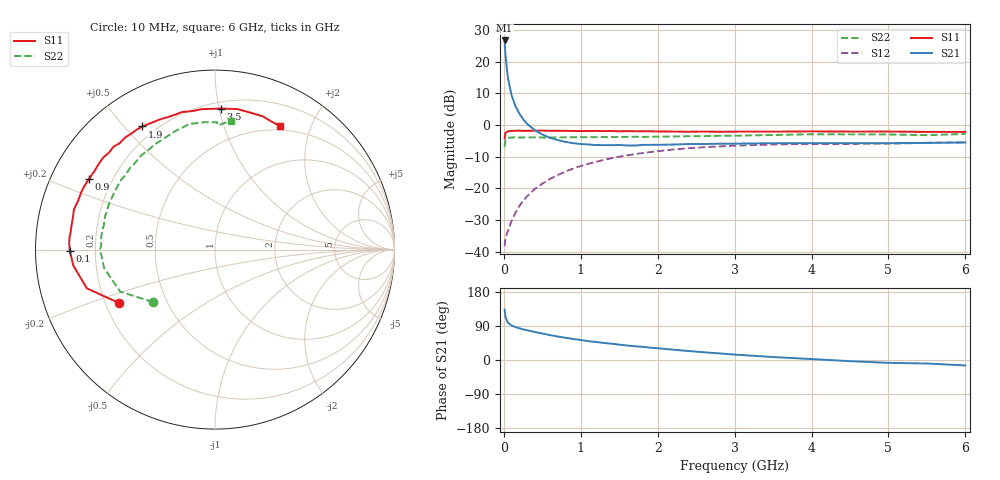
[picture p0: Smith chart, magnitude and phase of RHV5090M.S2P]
! SIEMENS Small Signal Semiconductors
! BFR106
! Si NPN RF Bipolar Junction Transistor in SOT23
! VCE = 0.5 V  IC = 90 mA
! Common Emitter S-Parameters:  August  1996
# GHz  S  MA  R  50
!  f  S11  S21  S12  S22
! GHz  MAG  ANG  MAG  ANG  MAG  ANG  MAG  ANG
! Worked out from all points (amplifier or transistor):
!   36 points, 10 MHz to 6 GHz, reference 50 ohm
!   highest |S21| = 26.7 dB at 10 MHz (marker M1)
!   |S21| within 3 dB of that: start of sweep to 17.19 MHz
!   unconditionally stable (mu >= 1): start of sweep to 17.92 MHz; 25.4 MHz to end of sweep
!   at 250 MHz: K = 1.83, MAG = 7.6 dB, |S12| = -24.0 dB
!   at 1.4 GHz: K = 1.30, MAG = -1.2 dB, |S12| = -10.5 dB
!   at 6 GHz: K = 1.03, MAG = -1.2 dB, |S12| = -5.5 dB
!   S11 on the Smith chart (normalised r, x): 10 MHz: 0.26, -0.24; 100 MHz: 0.11, -0.00; 900 MHz: 0.12, +0.26; 1.9 GHz: 0.15, +0.56; 3.5 GHz: 0.25, +1.01; 6 GHz: 0.45, +1.57
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0.01  0.6129 -151.0  21.66 133.3  0.0122 45.1  0.4519 -139.7
0.02  0.7461 -163.2  13.4 114.9  0.016 37.1  0.578 -156.1
0.05  0.7944 -173.6  5.837 98.9  0.0209 44.4  0.6261 -170.4
0.1  0.8092 -179.6  2.967 91.1  0.0305 56.9  0.6343 -177.4
0.15  0.813 177.3  2.003 86.9  0.0409 62.6  0.6416 -179.8
0.2  0.8134 175.1  1.526 83.8  0.0522 66.2  0.6341 177.9
0.25  0.8101 173.0  1.236 80.9  0.0634 67.6  0.637 176.1
0.3  0.8106 170.8  1.05 78.7  0.0747 68.5  0.6376 174.8
0.4  0.8117 167.2  0.833 74.0  0.0968 68.7  0.6377 172.2
0.5  0.817 164.2  0.71 69.9  0.1185 68.0  0.636 169.7
0.6  0.81 160.3  0.627 65.6  0.1408 66.6  0.6339 167.5
0.9  0.8048 150.8  0.517 55.5  0.2049 61.1  0.6394 160.4
1.1  0.8044 143.7  0.493 49.6  0.2443 57.0  0.6434 156.3
1.5  0.796 131.9  0.484 40.5  0.3159 48.1  0.6479 147.3
1.9  0.7965 120.5  0.486 32.6  0.3734 39.5  0.6518 138.6
2.2  0.7879 113.3  0.492 27.3  0.4095 33.3  0.6577 132.0
2.8  0.7819 99.2  0.507 17.4  0.459 22.1  0.6754 120.3
3.5  0.7867 87.5  0.516 7.8  0.4928 11.1  0.696 108.8
4.5  0.788 75.1  0.517 -3.1  0.5049 -1.4  0.7123 94.9
5  0.7884 70.2  0.517 -7.5  0.5078 -6.2  0.7096 89.1
5.5  0.7793 65.8  0.522 -9.2  0.5226 -8.5  0.692 88.6
6  0.7781 62.1  0.53 -14.4  0.5338 -14.1  0.7231 83.1
